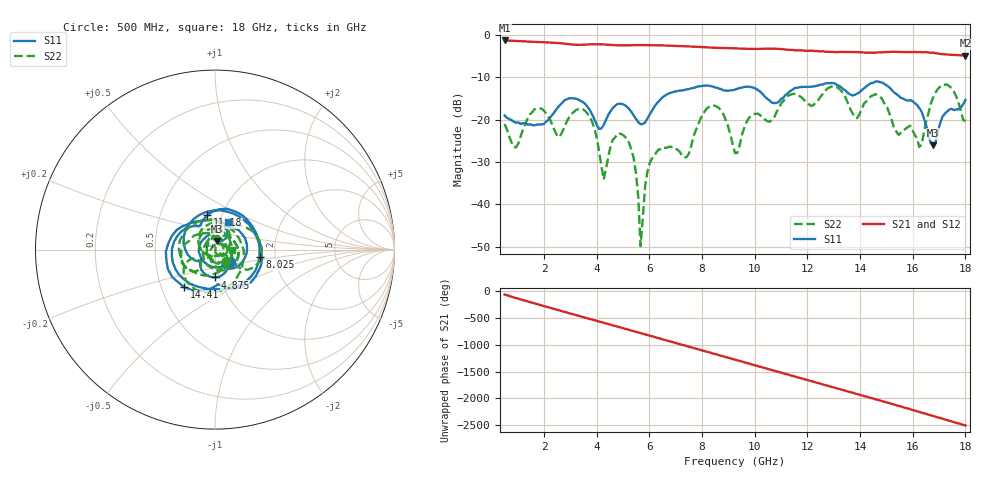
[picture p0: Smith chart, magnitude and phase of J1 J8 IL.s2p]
!Agilent Technologies,N5230A,MY45001360,A.07.50.67
!Agilent N5230A: A.07.50.67
!Date: Tuesday, April 16, 2024 17:49:30
!Correction: S11(Full 2 Port(1,2))
!S21(Full 2 Port(1,2))
!S12(Full 2 Port(1,2))
!S22(Full 2 Port(1,2))
!S2P File: Measurements: S11, S21, S12, S22:
# Hz S  dB  R 50
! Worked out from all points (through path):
!   201 points, 500 MHz to 18 GHz, reference 50 ohm
!   highest |S21| = -1.28 dB at 500 MHz (marker M1); lowest = -4.9 dB at 18 GHz (marker M2)
!   group delay of S21, straight-line fit = 386 ps
!   lowest |S11| = -26.0 dB at 16.77 GHz (marker M3), VSWR 1.11, Z = 50.9 + j4.97 ohm
!   |S11| at or under -10 dB: start of sweep to end of sweep
!   |S22| runs from -49.8 to -11.7 dB; largest |S21 - S12| = 0.007
!   S11 on the Smith chart (normalised r, x): 500 MHz: 1.18, -0.17; 4.875 GHz: 0.95, -0.30; 8.025 GHz: 1.65, -0.14; 11.18 GHz: 0.85, +0.34; 14.41 GHz: 0.66, -0.30; 18 GHz: 1.10, +0.35
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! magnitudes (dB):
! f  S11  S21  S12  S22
! 500 MHz  -19.0  -1.3  -1.3  -21.0
! 937.5 MHz  -20.7  -1.4  -1.4  -26.5
! 1.637 GHz  -21.3  -1.6  -1.6  -17.5
! 2.513 GHz  -17.2  -1.9  -1.9  -24.0
! 3.475 GHz  -15.8  -2.3  -2.3  -17.5
! 4.263 GHz  -21.3  -2.2  -2.2  -34.1
! 4.875 GHz  -16.2  -2.4  -2.4  -23.3
! 5.4 GHz  -18.9  -2.4  -2.4  -29.0
! 5.662 GHz  -21.1  -2.4  -2.4  -49.8
! 5.925 GHz  -19.7  -2.4  -2.4  -32.2
! 6.362 GHz  -15.6  -2.4  -2.4  -26.9
! 7.412 GHz  -12.8  -2.7  -2.7  -28.8
! 8.025 GHz  -12.0  -2.9  -2.8  -18.8
! 8.725 GHz  -12.8  -3.0  -3.0  -17.8
! 9.25 GHz  -12.9  -3.1  -3.1  -27.9
! 11.18 GHz  -14.1  -3.4  -3.4  -15.0
! 12.22 GHz  -12.1  -3.7  -3.7  -16.6
! 14.41 GHz  -11.4  -4.2  -4.2  -14.5
! 15.11 GHz  -12.4  -4.0  -4.0  -18.5
! 16.25 GHz  -17.2  -4.0  -4.0  -26.4
! 16.77 GHz  -26.0  -4.2  -4.2  -14.8
! 18 GHz  -15.3  -4.9  -4.9  -20.3
